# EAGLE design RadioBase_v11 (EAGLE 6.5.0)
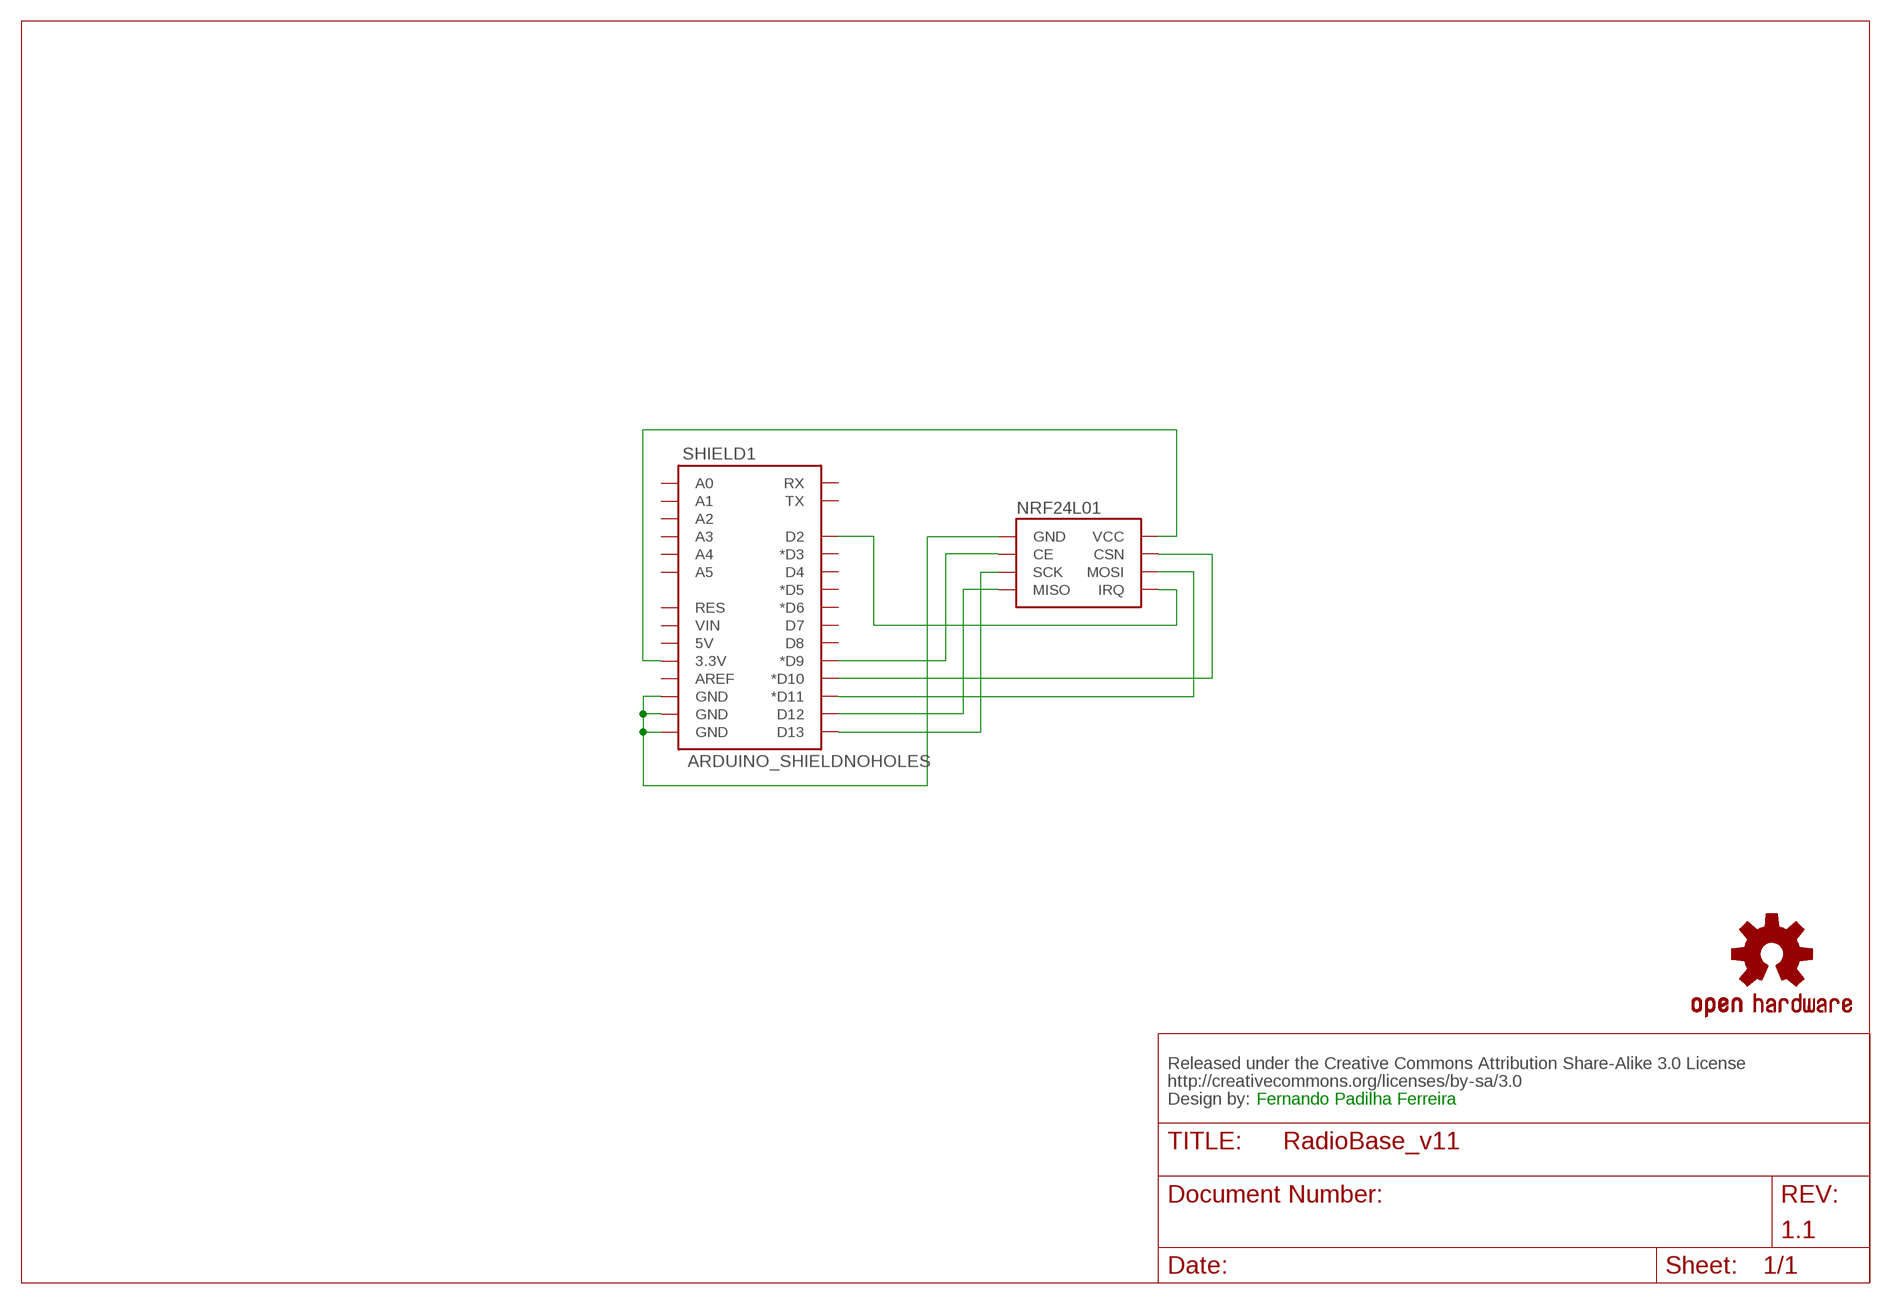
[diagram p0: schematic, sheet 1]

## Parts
CC_TEXT1  CREATIVE_COMMONS  [CREATIVE_COMMONS]
LOGO1  OSHW-LOGOL  [OSHW-LOGO-L]
NRF24L01  NRF24L01  [NRF24L01]
SHIELD1  ARDUINO_SHIELDNOHOLES  [DUEMILANOVE_SHIELD_NOHOLES]

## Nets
GND: NRF24L01.1(GND) SHIELD1.GND@0(GND) SHIELD1.GND@1(GND) SHIELD1.GND@2(GND)
N$9: NRF24L01.3(CE) SHIELD1.D9(*D9)
N$10: NRF24L01.4(CSN) SHIELD1.D10(*D10)
N$11: NRF24L01.6(MOSI) SHIELD1.D11(*D11)
N$12: NRF24L01.7(MISO) SHIELD1.D12
N$13: NRF24L01.5(SCK) SHIELD1.D13
N$14: NRF24L01.2(VCC) SHIELD1.3.3V
NRF24L02: NRF24L01.8(IRQ) SHIELD1.D2
Unconnected: SHIELD1.5V SHIELD1.A0 SHIELD1.A1 SHIELD1.A2 SHIELD1.A3 SHIELD1.A4 SHIELD1.A5 SHIELD1.AREF SHIELD1.D3(*D3) SHIELD1.D4 SHIELD1.D5(*D5) SHIELD1.D6(*D6) SHIELD1.D7 SHIELD1.D8 SHIELD1.RES SHIELD1.RX SHIELD1.TX SHIELD1.VIN

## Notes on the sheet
- Fernando Padilha Ferreira
- 1.1

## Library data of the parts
CC_TEXT1 = SparkFun-Aesthetics:CREATIVE_COMMONS: Creative Commons License summary
LOGO1 = SparkFun-Aesthetics:OSHW-LOGO: Open Source Hardware Logo This logo indicates the piece of hardware it is found on incorporates a OSHW license and/or adheres to the definition of open source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
NRF24L01 = microbuilder:NRF24L01: TRANSCEIVER / TRANSCEPTOR NRF24L01
SHIELD1 = SparkFun-Boards:ARDUINO_SHIELD: Arduino shield footprint

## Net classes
0 default: width 0.305 mm
2 gnd: width 0.305 mm, drill 0.559 mm, clearance 0.254 mm

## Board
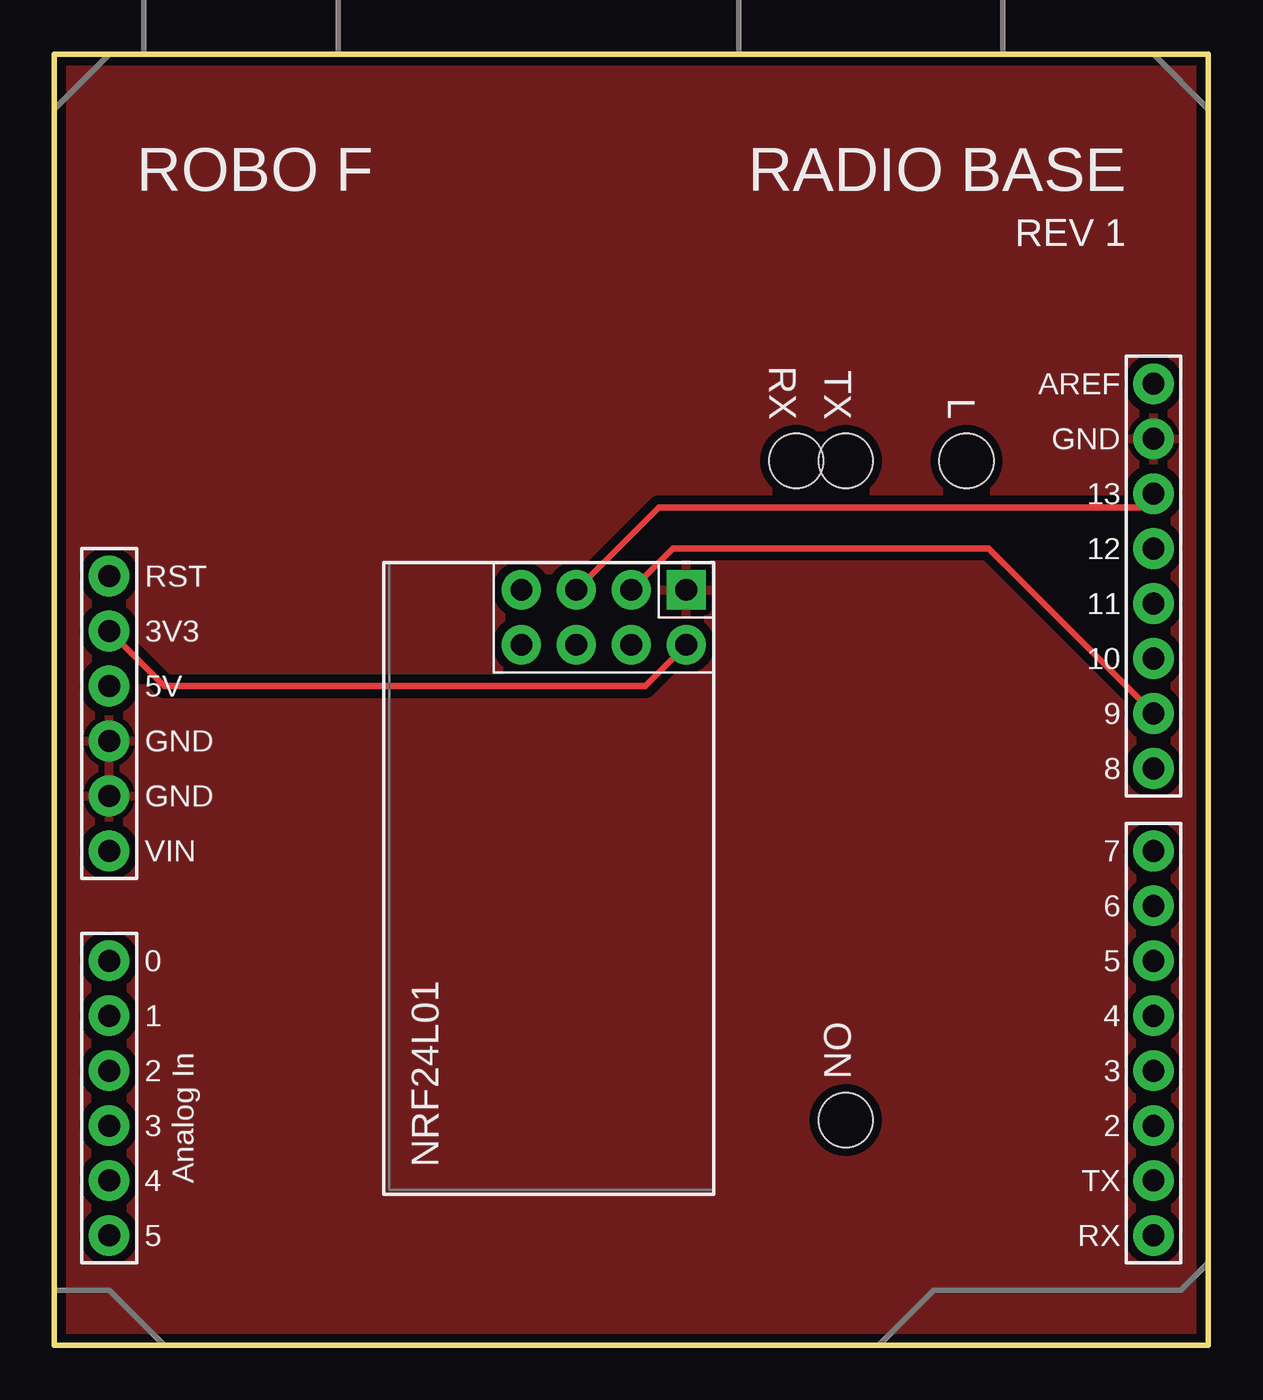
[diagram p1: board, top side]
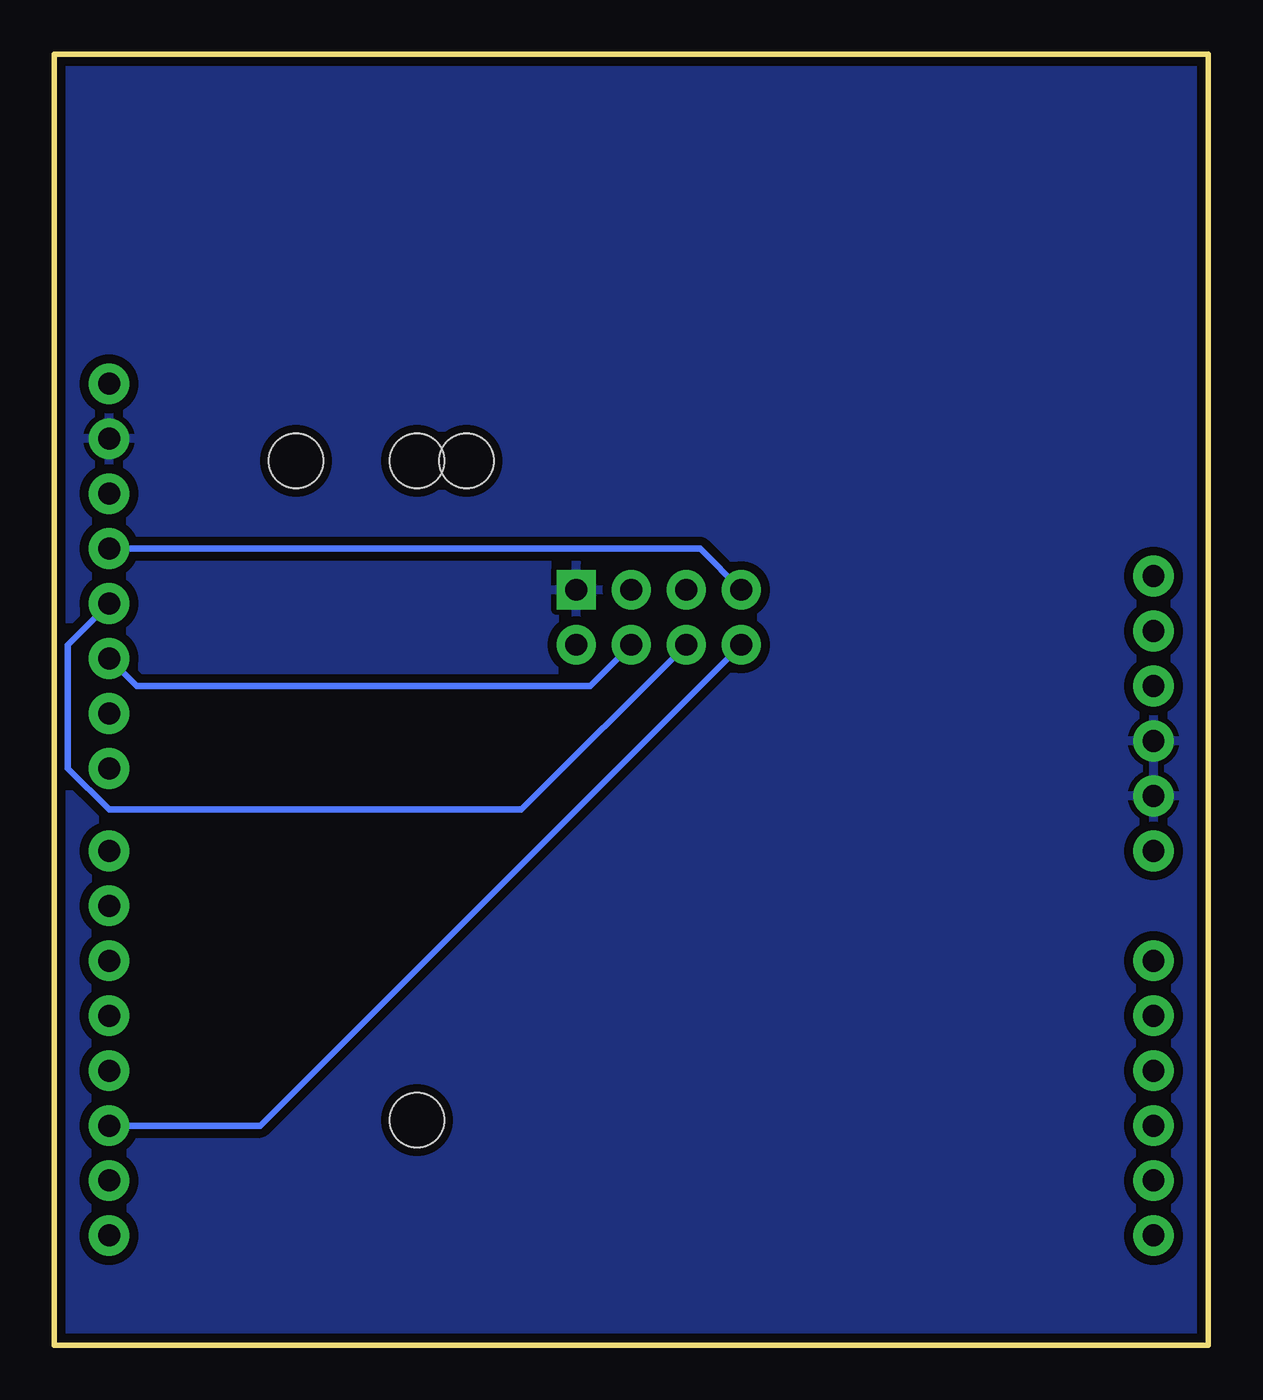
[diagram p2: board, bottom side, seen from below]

Size 53.34 x 59.69 mm. Coordinates in mm from the lower left corner, seen from the top.
Outline: 0,0 53.34,0 53.34,59.69 0,59.68 0,0
Copper layers (1*16): Top 0.035mm / dielectric 1.5mm / Bottom 0.035mm
Design rules "peteco *": minimum track width 12mil, minimum drill 19mil, track to track 10mil, track to pad 10mil, pad to pad 10mil, via to via 10mil, smd to smd 0mil, copper to edge 10mil, drill to drill 8mil, minimum pad ring 16mil, minimum via ring 8mil, stop-mask expansion 4mil, vias tented up to drill 0mil, thermal gap 10mil
Holes 2.5 mm at 34.29,40.89 36.58,40.89 42.16,40.89 36.58,10.41

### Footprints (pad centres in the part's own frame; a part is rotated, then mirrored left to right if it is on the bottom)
NRF24L01 = drill 1 square: 1 -1.27,1.27 | drill 1: 2 -3.81,1.27; 3 -1.27,3.81; 4 -3.81,3.81; 5 -1.27,6.35; 6 -3.81,6.35; 7 -1.27,8.89; 8 -3.81,8.89
DUEMILANOVE_SHIELD_NOHOLES = drill 1.016 pad 1.88: 3.3V 50.8,26.67; 5V 50.8,29.21; A0 50.8,41.91; A1 50.8,44.45; A2 50.8,46.99; A3 50.8,49.53; A4 50.8,52.07; A5 50.8,54.61; AREF 2.54,15.24; D2 2.54,49.53; D3 2.54,46.99; D4 2.54,44.45; D5 2.54,41.91; D6 2.54,39.37; D7 2.54,36.83; D8 2.54,33.02; D9 2.54,30.48; D10 2.54,27.94; D11 2.54,25.4; D12 2.54,22.86; D13 2.54,20.32; GND@0 50.8,31.75; GND@1 50.8,34.29; GND@2 2.54,17.78; RES 50.8,24.13; RX 2.54,54.61; TX 2.54,52.07; VIN 50.8,36.83

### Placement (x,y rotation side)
CC_TEXT1  not placed on the board
LOGO1  not placed on the board
NRF24L01  30.48,36.2 90 top
SHIELD1  53.34,59.69 180 top

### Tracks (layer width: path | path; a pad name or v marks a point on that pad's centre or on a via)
GND
  pour Top (isolate 0.406): 0,0 53.34,0 53.34,59.69 0,59.69
  pour Bottom (isolate 0.406): 0,0 53.34,0 53.34,59.69 0,59.69
N$9
  Top 0.305: NRF24L01.3 28.57,36.83 43.18,36.83 SHIELD1.D9
N$10
  Bottom 0.305: NRF24L01.4 28.57,30.48 49.53,30.48 SHIELD1.D10
N$11
  Bottom 0.305: NRF24L01.6 31.75,24.77 50.8,24.77 52.7,26.67 52.7,32.38 SHIELD1.D11
N$12
  Bottom 0.305: NRF24L01.7 23.5,36.83 SHIELD1.D12
N$13
  Top 0.305: NRF24L01.5 27.94,38.73 50.16,38.73 SHIELD1.D13
N$14
  Top 0.305: NRF24L01.2 27.3,30.48 5.08,30.48 SHIELD1.3.3V
NRF24L02
  Bottom 0.305: NRF24L01.8 43.81,10.16 SHIELD1.D2

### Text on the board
tPlace: ROBO F | RADIO BASE | REV 1 | RX | TX | L | ON
tDocu: Fernando Padilha Ferreira

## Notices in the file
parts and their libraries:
SparkFun-Boards: Licensing: CC v3.0 Share-Alike You are welcome to use this library for commercial purposes.
SparkFun-Aesthetics: Released under the Creative Commons Attribution Share-Alike 3.0 License
SparkFun-Aesthetics: http://creativecommons.org/licenses/by-sa/3.0
